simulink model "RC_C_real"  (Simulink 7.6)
settings: Solver=ode23t  StartTime=0.0  StopTime=0.12  RelTol=1e-3
InitFcn:
  | R=1e3;
  | C=10e-6;
StopFcn:
  | close all
  | load VC_circuit_RC.mat
  | plot(x(1,:),x(2,:))
  | hold on
  | plot(x(1,:),x(3,:))
  | axis([0 0.12 -0.2 1.2])
  | grid
  | title('Tension aux bornes de C et créneau d''entrée')
  | ylabel('Circuit RC - Simulation de la capacité')
  | xlabel('temps')
libraries: powerlib x7, powerlib_extras x1

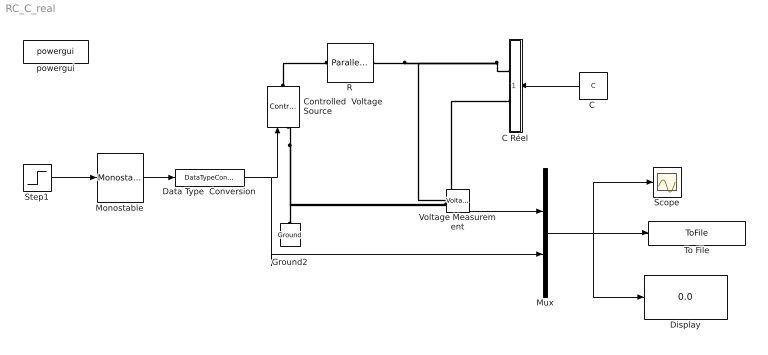
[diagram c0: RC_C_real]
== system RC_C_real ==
  "C " : Constant  Value=C
  C Réel : Subsystem
  Controlled  Voltage Source : powerlib/Electrical Sources/Controlled Voltage Source  DialogController=POWERSYS.PowerSysDialog  SystemSampleTime=-1  Initialize=on  Source_Type=AC  Amplitude=0  Phase=0  Frequency=0  Measurements=None
  Data Type  Conversion : DataTypeConversion  OutDataTypeStr=double
  Display : Display
  Ground2 : powerlib/Elements/Ground  DialogController=POWERSYS.PowerSysDialog  PhysicalDomain=powersysdomain  SubClassName=unknown  LeftPortType=p1  RightPortType=p1  LConnTagsString=a
  Monostable : powerlib_extras/Control  Blocks/Monostable  DialogController=POWERSYS.PowerSysDialog  SystemSampleTime=-1  EdgeDetect=Either  t_mono=0.06  ic=0
  Mux : Mux  Inputs=2
  R : powerlib/Elements/Parallel RLC Branch  DialogController=POWERSYS.PowerSysDialog  PhysicalDomain=powersysdomain  SubClassName=unknown  LeftPortType=p1  RightPortType=p1  LConnTagsString=a  RConnTagsString=__new0  BranchType=R  Resistance=R  Inductance=10e-03  SetiL0=off  InitialCurrent=0  Capacitance=[]  Setx0=off  InitialVoltage=0  Measurements=None
  Scope : Scope
  Step1 : Step  Time=0.01  SampleTime=0
  To File : ToFile  Filename=VC_circuit_RC  MatrixName=x
  Voltage Measurement : powerlib/Measurements/Voltage Measurement  DialogController=POWERSYS.PowerSysDialog  SystemSampleTime=-1  PhasorSimulation=off  OutputType=Complex  PSBequivalent=0
  powergui : powerlib/powergui  SystemSampleTime=-1  SimulationMode=Continuous  SampleTime=0  frequency=60  SPID=off  DisableSnubberDevices=off  DisableRonSwitches=off  DisableVfSwitches=off  SwTol=0  Interpol=off  frequencyindice=0  echomessages=off  HookPort=off  DisplayEquations=off  FunctionMessages=off  EnableUseOfTLC=off  x0status=blocks  RestoreLinks=warning  ResistiveCurrentMeasurement=off  Frange=[0:2:500]  Ylog=off  Xlog=on  ShowGrid=off  save=off  variable=ZData  ZoomFFT=on  StartTime=0.0  cycles=1  DisplayStyle=1  fundamental=60  FreqAxis=off  MaxFrequency=1000  frequencyindicesteady=60  RmsSteady=1  display=off  Ts=0  methode=off
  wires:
  Step1/1 -> Monostable/1
  Monostable/1 -> Data Type  Conversion/1
  Data Type  Conversion/1 -> Controlled  Voltage Source/1, Mux/2
  Voltage Measurement/1 -> Mux/1
  Mux/1 -> Scope/1, To File/1, Display/1
  "C "/1 -> C Réel/1(C)
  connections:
  C Réel/RConn2 -- Controlled  Voltage Source/LConn1 -- Ground2/LConn1 -- Voltage Measurement/LConn2
  C Réel/RConn1 -- Voltage Measurement/LConn1 -- R/LConn1
  Controlled  Voltage Source/RConn1 -- R/RConn1

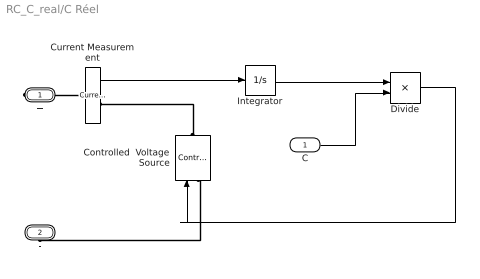
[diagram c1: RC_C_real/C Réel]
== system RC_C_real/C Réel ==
  C : Inport
  Controlled  Voltage Source : powerlib/Electrical Sources/Controlled Voltage Source  DialogController=POWERSYS.PowerSysDialog  SystemSampleTime=-1  Initialize=on  Source_Type=AC  Amplitude=0  Phase=0  Frequency=0  Measurements=None
  Current Measurement : powerlib/Measurements/Current Measurement  DialogController=POWERSYS.PowerSysDialog  SystemSampleTime=-1  PhasorSimulation=off  OutputType=Complex  PSBequivalent=0
  Divide : Product  Inputs=*/
  Integrator : Integrator
  + : PMIOPort  Port=1  Side=Right
  - : PMIOPort  Port=2  Side=Right
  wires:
  C/1 -> Divide/2
  Integrator/1 -> Divide/1
  Current Measurement/1 -> Integrator/1
  Divide/1 -> Controlled  Voltage Source/1
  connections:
  -/RConn1 -- Controlled  Voltage Source/LConn1
  +/RConn1 -- Current Measurement/LConn1
  Controlled  Voltage Source/RConn1 -- Current Measurement/RConn1
